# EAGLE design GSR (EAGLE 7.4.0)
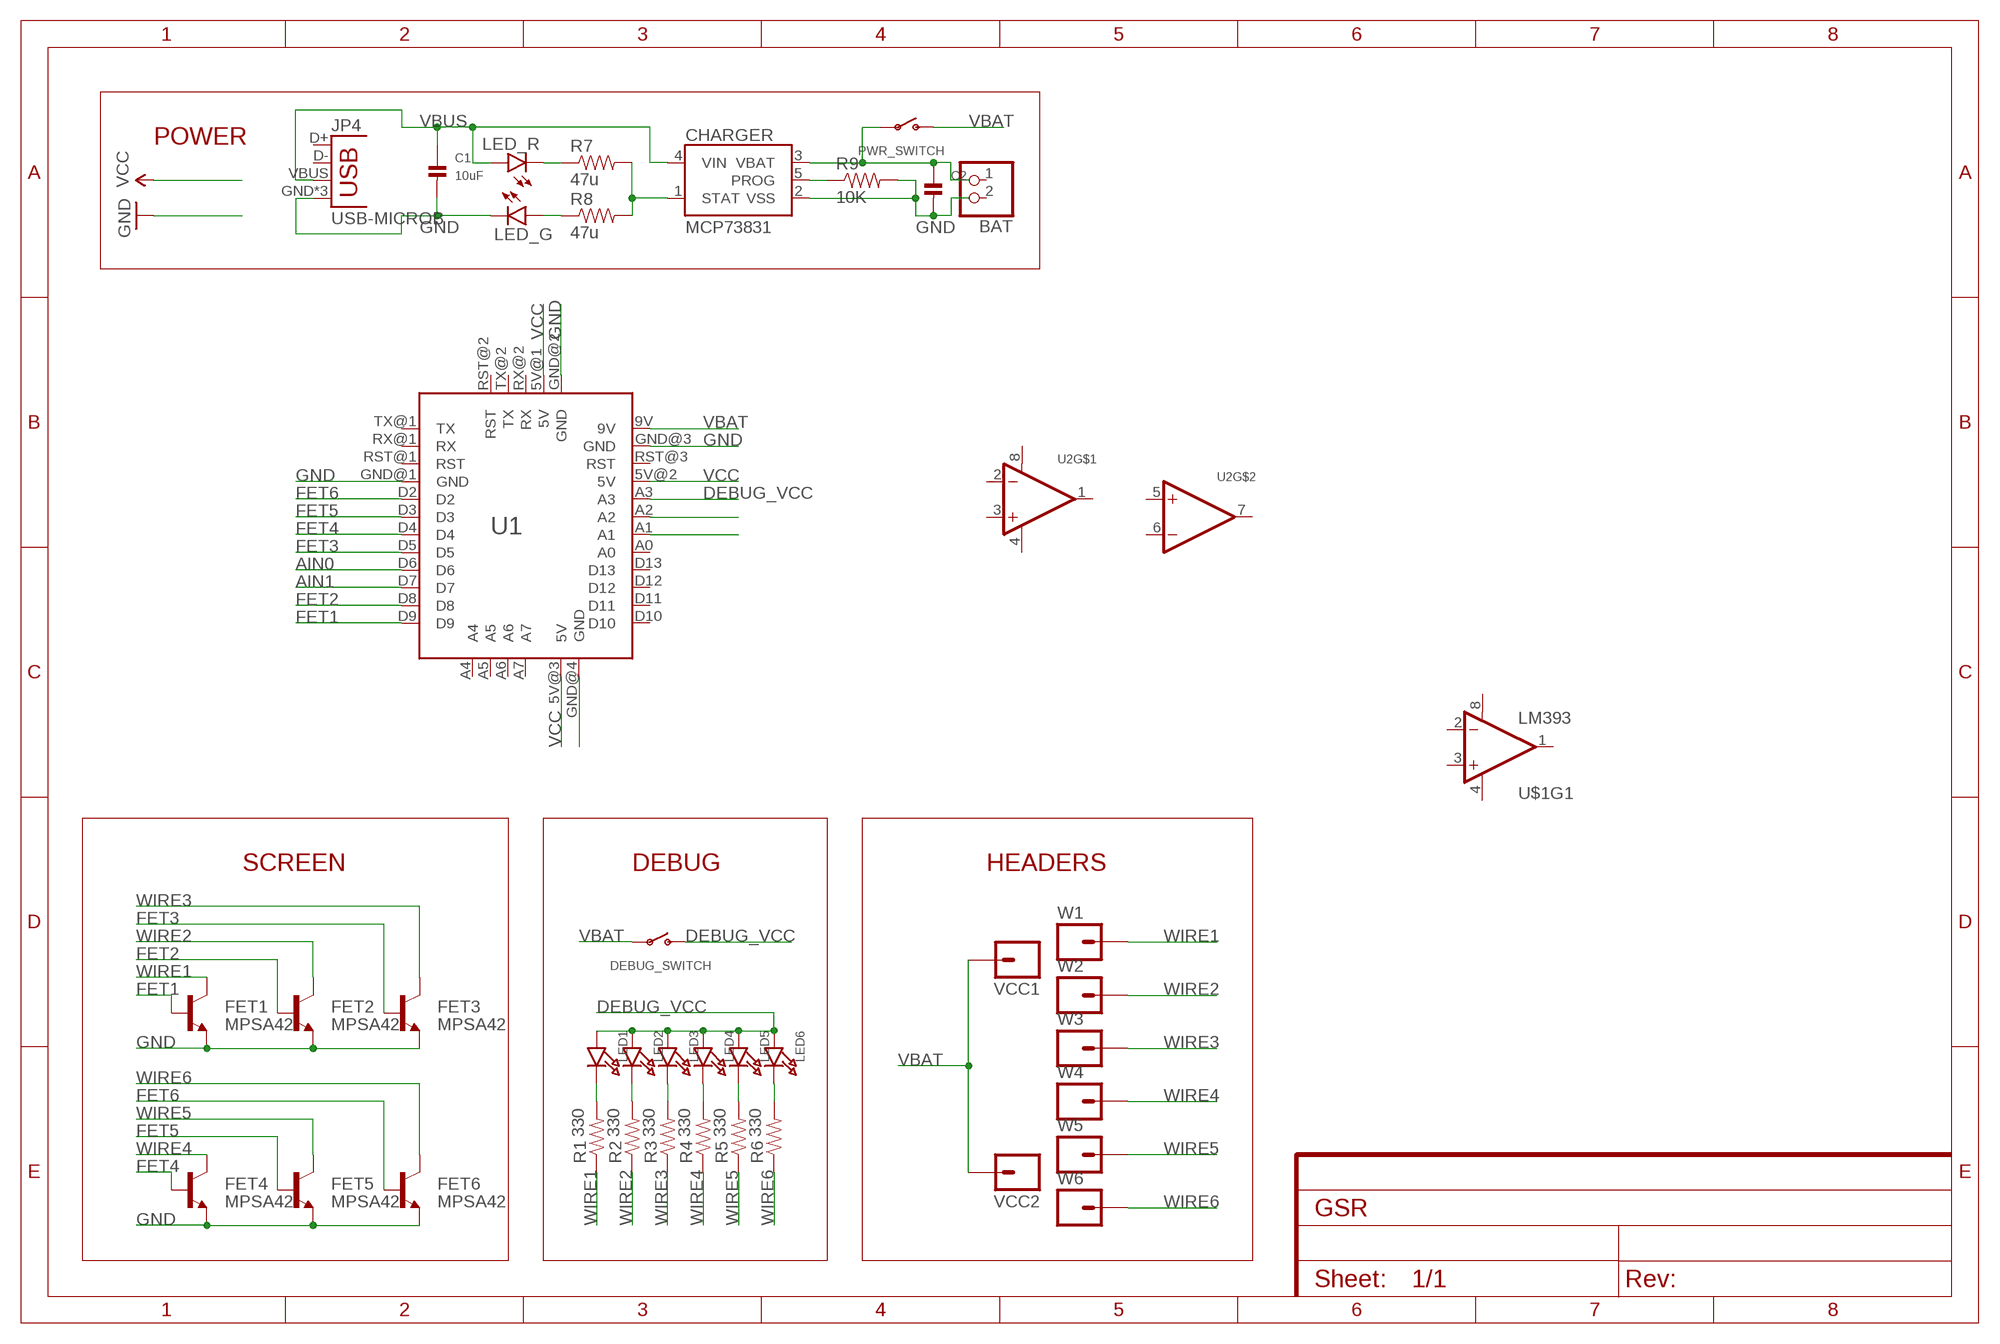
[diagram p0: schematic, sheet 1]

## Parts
BAT  JST_2PIN-SMT  [JST-PH-2-SMT]
C1  10uF  CAP_CERAMIC0603  [0603]
C2  CAP_CERAMIC0603  [0603]
CHARGER  MCP73831  [SOT23-5]
DEBUG_SWITCH  SWITCH_SPST  [SPST_SMT_19192]
FET1  MPSA42  TRANSISTOR_NPNMPSA42  [SOT23-3]
FET2  MPSA42  TRANSISTOR_NPNMPSA42  [SOT23-3]
FET3  MPSA42  TRANSISTOR_NPNMPSA42  [SOT23-3]
FET4  MPSA42  TRANSISTOR_NPNMPSA42  [SOT23-3]
FET5  MPSA42  TRANSISTOR_NPNMPSA42  [SOT23-3]
FET6  MPSA42  TRANSISTOR_NPNMPSA42  [SOT23-3]
JP4  USB-MICROB  [USB-MICROB]
LED1  LED0603_NOOUTLINE  [CHIPLED_0603_NOOUTLINE]
LED2  LED0603_NOOUTLINE  [CHIPLED_0603_NOOUTLINE]
LED3  LED0603_NOOUTLINE  [CHIPLED_0603_NOOUTLINE]
LED4  LED0603_NOOUTLINE  [CHIPLED_0603_NOOUTLINE]
LED5  LED0603_NOOUTLINE  [CHIPLED_0603_NOOUTLINE]
LED6  LED0603_NOOUTLINE  [CHIPLED_0603_NOOUTLINE]
LED_G  LED0603  [LED-0603]
LED_R  LED0603  [LED-0603]
PWR_SWITCH  SWITCH_SPST  [SPST_SMT_19192]
R1  330  RESISTOR0603-RES  [0603-RES]
R2  330  RESISTOR0603-RES  [0603-RES]
R3  330  RESISTOR0603-RES  [0603-RES]
R4  330  RESISTOR0603-RES  [0603-RES]
R5  330  RESISTOR0603-RES  [0603-RES]
R6  330  RESISTOR0603-RES  [0603-RES]
R7  47u  RESISTOR0603  [0603-RES]
R8  47u  RESISTOR0603  [0603-RES]
R9  10K  RESISTOR0603  [0603-RES]
U1  ARDUINO_MINI  [ARDUINO_MINI]
U2  OPAMP_DUALMSOP8_65  [MSOP8_0.65MM]
U$1  LM393  [SO08]
VCC1  M01NOSILK-KIT  [1X01NS-KIT]
VCC2  M01NOSILK-KIT  [1X01NS-KIT]
W1  M01NOSILK-KIT  [1X01NS-KIT]
W2  M01NOSILK-KIT  [1X01NS-KIT]
W3  M01NOSILK-KIT  [1X01NS-KIT]
W4  M01NOSILK-KIT  [1X01NS-KIT]
W5  M01NOSILK-KIT  [1X01NS-KIT]
W6  M01NOSILK-KIT  [1X01NS-KIT]

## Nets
AIN0: U1.D6
AIN1: U1.D7
DEBUG_VCC: DEBUG_SWITCH.C(S) LED1.A LED2.A LED3.A LED4.A LED5.A LED6.A U1.A3
FET1: FET1.1(B) U1.D9
FET2: FET2.1(B) U1.D8
FET3: FET3.1(B) U1.D5
FET4: FET4.1(B) U1.D4
FET5: FET5.1(B) U1.D3
FET6: FET6.1(B) U1.D2
GND: C1.2 C2.2 CHARGER.2(VSS) FET1.2(E) FET2.2(E) FET3.2(E) FET4.2(E) FET5.2(E) FET6.2(E) JP4.GND JP4.MT1(GND) JP4.MT2(GND) LED_G.C R9.2 U1.GND@1(GND) U1.GND@2(GND) U1.GND@3(GND) U1.GND@4(GND)
N$1: LED1.C R1.2
N$2: LED2.C R2.2
N$3: LED3.C R3.2
N$4: LED4.C R4.2
N$5: LED5.C R5.2
N$6: LED6.C R6.2
N$7: CHARGER.1(STAT) R7.2 R8.2
N$10: LED_G.A R8.1
N$11: LED_R.C R7.1
N$14: CHARGER.5(PROG) R9.1
N$36: U1.A2
N$37: U1.A1
VBAT: DEBUG_SWITCH.B(P) PWR_SWITCH.C(S) U1.9V VCC1.1 VCC2.1
VBAT_IN: C2.1 CHARGER.3(VBAT) PWR_SWITCH.B(P)
VBUS: C1.1 CHARGER.4(VIN) JP4.VBUS LED_R.A
VCC: U1.5V@1(5V) U1.5V@2(5V) U1.5V@3(5V)
WIRE1: FET1.3(C) R1.1 W1.1
WIRE2: FET2.3(C) R2.1 W2.1
WIRE3: FET3.3(C) R3.1 W3.1
WIRE4: FET4.3(C) R4.1 W4.1
WIRE5: FET5.3(C) R5.1 W5.1
WIRE6: FET6.3(C) R6.1 W6.1
Unconnected: BAT.1 BAT.2 JP4.D+ JP4.D- U1.A0 U1.A4 U1.A5 U1.A6 U1.A7 U1.D10 U1.D11 U1.D12 U1.D13 U1.RST@1(RST) U1.RST@2(RST) U1.RST@3(RST) U1.RX@1(RX) U1.RX@2(RX) U1.TX@1(TX) U1.TX@2(TX) U2.1(OUT) U2.2(-IN) U2.3(+IN) U2.5(+IN) U2.6(-IN) U2.7(OUT) U$1.1(OUT) U$1.2(-IN) U$1.3(+IN) U$1.5(+IN) U$1.6(-IN) U$1.7(OUT)

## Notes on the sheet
- POWER
- SCREEN | DEBUG | HEADERS

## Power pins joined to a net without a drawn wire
V+: U2.8(V+) U$1.8(V+)
V-: U2.4(V-) U$1.4(V-)

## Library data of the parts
BAT = adafruit:JST_2PIN: JST 2-Pin Connectors of various flavors
C1 C2 = microbuilder:CAP_CERAMIC: Ceramic Capacitors
CHARGER = SparkFun-PowerIC:MCP73831: Miniature single cell, fully integrated Li-Ion, Li-polymer charge management controller http://ww1.microchip.com/downloads/en/DeviceDoc/20001984g.pdf IC-09995; PROD_ID: IC-09995
DEBUG_SWITCH PWR_SWITCH = microbuilder:SWITCH_SPST: Switch - SPST
FET1-FET6 = SparkFun-DiscreteSemi:TRANSISTOR_NPN: Generic NPN BJT MMBT2222A - TRANS-08049 (SOT-23, 1A 40V) MPSA42 - TRANS-09116 (SOT-23, 500mA 300V) MMBT5088LT1G - TRANS-11160 (SOT-23, 50 mA 30V) BC547 - COM-08928 (TO-92 45V 100mA) (1.Collector 2.Base 3.Emitter) 2N3904 - COM-00521 (TO-92 40V 200mA) (1.Emitter 2.Base 3.Collector) P2N2222A -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; PROD_ID: TRANS-09116
JP4 = SparkFun-Connectors:USB: USB Connectors USB-B-PTH is fully proven SKU : PRT-00139/CONN-08278 USB-miniB is fully proven SKU : PRT-00587 USB-A-PCB is untested. USB-A-H is throughly reviewed, but untested. Spark Fun Electronics SKU : PRT-00437 USB-B-SMT is throughly reviewed, but untested. Needs silkscreen touching up.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; PROD_ID: CONN-09505
LED1-LED6 = microbuilder:LED: LED
LED_G LED_R = SparkFun-LED:LED: LEDs
R1-R6 = SparkFun-Passives:RESISTOR: Resistor
R7-R9 = SparkFun-Resistors:RESISTOR: Resistor
U1 = myParts:ARDUINO_MINI: Arduino Mini V5 Footprint
U2 = microbuilder:OPAMP_DUAL: Dual Op-Amp MSOP8 - 0.65mm Pitch Manuf. ID Slew Rate Gain Bandwidth Prod. -3dB Bandwidth Current Input Bias Voltage Input Offset Supply - Single Supply - Dual Digikey Mouser EL5236IYZ-T7 128V/µs 300MHz 250MHz 6.5µA 100µV 5-12V +/-2.5-6V EL5236IYZ-T7TR-ND --
U$1 = SparkFun-AnalogIC:LM393: Low-voltage comparator
VCC1 VCC2 W1-W6 = SparkFun-Connectors:M01: Header 1

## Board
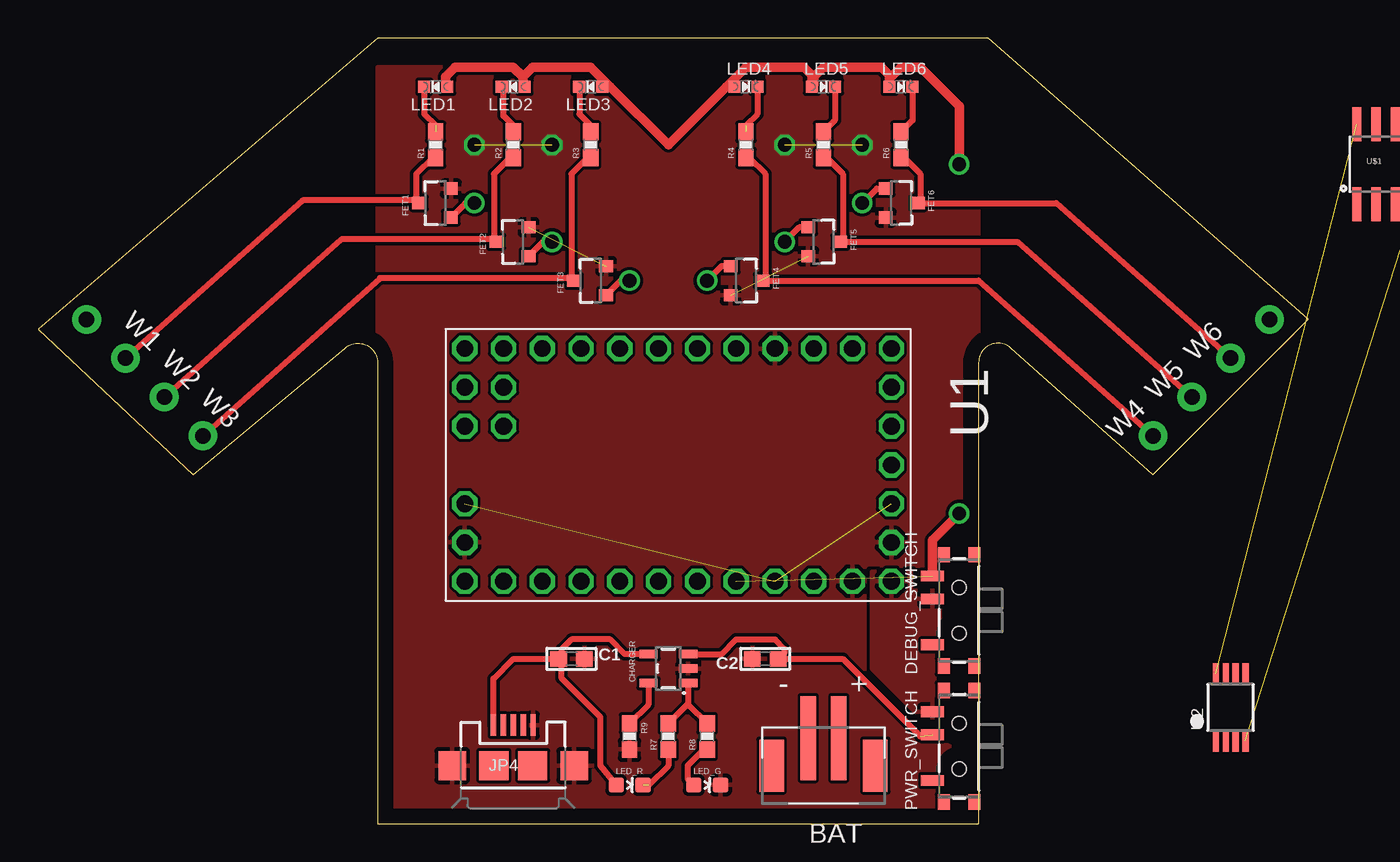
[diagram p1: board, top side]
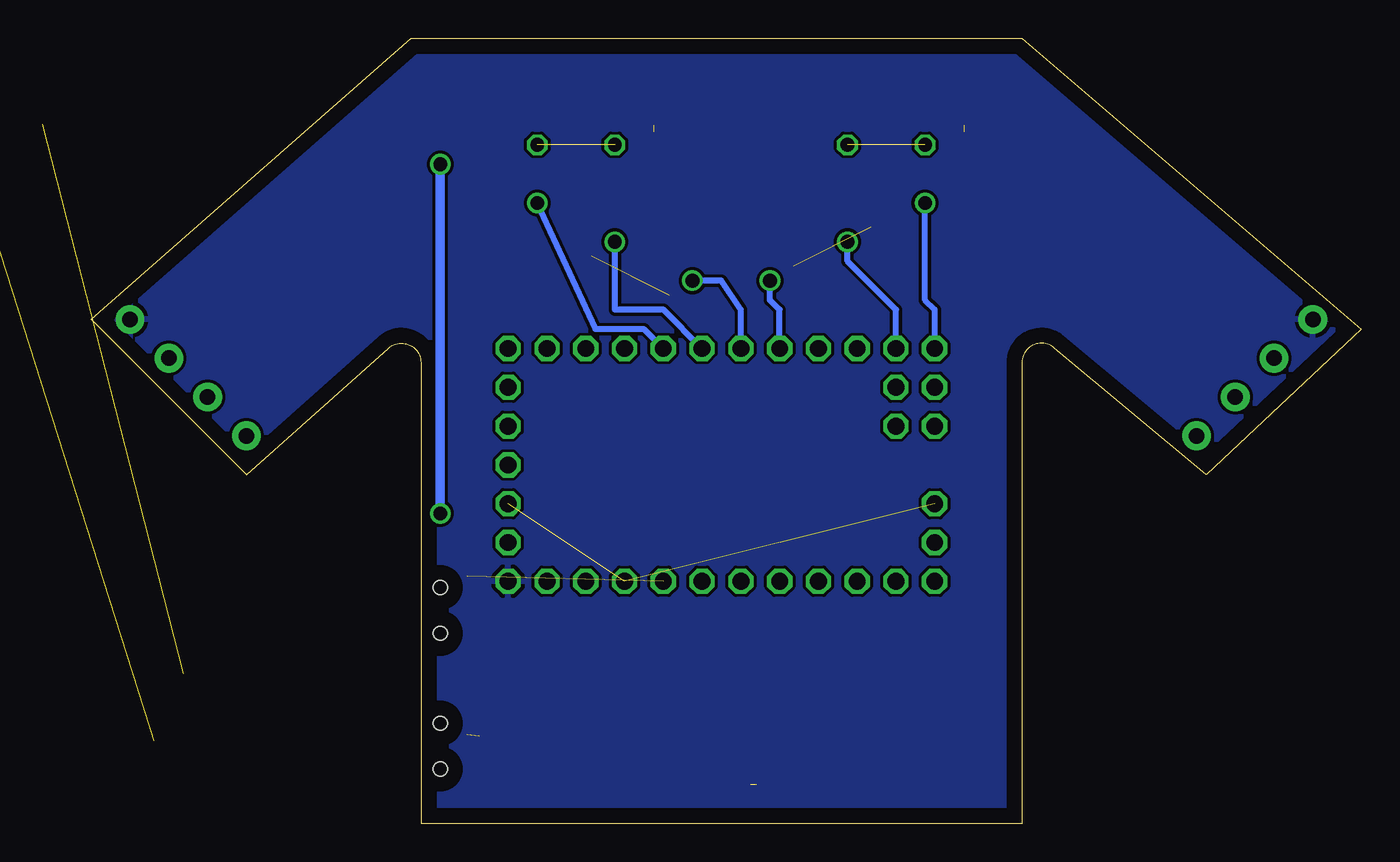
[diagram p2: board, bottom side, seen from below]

Size 83.19 x 51.44 mm. Coordinates in mm from the lower left corner, seen from the top.
Outline: 10.16,22.86 20.11,31.14 arc-132 22.22,30.19 22.22,0 61.59,0 61.59,30.19 arc-132 63.71,31.14 73.03,22.86 83.19,33.02 62.23,51.44 22.22,51.44 0,32.38 10.16,22.86
Copper layers (1*16): Top 0.035mm / dielectric 1.5mm / Bottom 0.035mm
Design rules "default": minimum track width 10mil, minimum drill 24mil, track to track 8mil, track to pad 8mil, pad to pad 8mil, via to via 8mil, smd to smd 8mil, copper to edge 40mil, drill to drill 8mil, minimum pad ring 10mil, minimum via ring 8mil, stop-mask expansion 4mil, vias tented up to drill 0mil, thermal gap 10mil

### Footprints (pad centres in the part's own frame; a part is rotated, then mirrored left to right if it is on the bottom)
JST-PH-2-SMT = smd 1 x 5.5: 1 -1,-1.8; 2 1,-1.8 | smd 1.6 x 3.4: NC1 -3.4,0; NC2 3.4,0
0603 = smd 1.1 x 1: 1 -0.85,0; 2 0.85,0
SOT23-5 = smd 0.55 x 1.2: 1 -0.95,-1.3; 2 0,-1.3; 3 0.95,-1.3; 4 0.95,1.3; 5 -0.95,1.3
SPST_SMT_19192 = smd 0.7 x 1.5: A -2.25,1.75; B 0.75,1.75; C 2.25,1.75 | smd 1 x 0.8: GND1 -3.65,1; GND2 -3.65,-1; GND3 3.65,1; GND4 3.65,-1 | hole 0.9: -1.5,0; 1.5,0
SOT23-3 = smd 0.8 x 0.9: 1 -0.95,-1; 2 0.95,-1; 3 0,1.1
USB-MICROB = smd 0.35 x 1.4: D+ 0,2.65; D- -0.65,2.65; GND 1.3,2.65; ID 0.65,2.65; VBUS -1.3,2.65 | smd 1.8 x 1.9: MT1 -4,0; MT2 4,0 | smd 1.9 x 1.9: P$1 -1.27,0; P$2 1.27,0
CHIPLED_0603_NOOUTLINE = smd 0.8 x 0.8: A 0,-0.75; C 0,0.75
LED-0603 = smd 1 x 1: A 0,-0.877; C 0,0.877
0603-RES = smd 1.1 x 1: 1 -0.85,0; 2 0.85,0
ARDUINO_MINI = drill 1.1 octagon: 5V@1 2.54,15.24; 5V@2 7.62,7.62; 5V@3 2.54,-12.7; 9V 7.62,15.24; A0 7.62,-2.54; A1 7.62,0; A2 7.62,2.54; A3 7.62,5.08; A4 -5.08,-12.7; A5 -2.54,-12.7; A6 -5.08,-10.16; A7 -2.54,-10.16; D2 -7.62,5.08; D3 -7.62,2.54; D4 -7.62,0; D5 -7.62,-2.54; D6 -7.62,-5.08; D7 -7.62,-7.62; D8 -7.62,-10.16; D9 -7.62,-12.7; D10 7.62,-12.7; D11 7.62,-10.16; D12 7.62,-7.62; D13 7.62,-5.08; GND@1 -7.62,7.62; GND@2 5.08,15.24; GND@3 7.62,12.7; GND@4 5.08,-12.7; RST@1 -7.62,10.16; RST@2 -5.08,15.24; RST@3 7.62,10.16; RX@1 -7.62,12.7; RX@2 0,15.24; TX@1 -7.62,15.24; TX@2 -2.54,15.24
MSOP8_0.65MM = smd 0.4 x 1.4: 1 -0.975,-2.2; 2 -0.325,-2.2; 3 0.325,-2.2; 4 0.975,-2.2; 5 0.975,2.2; 6 0.325,2.2; 7 -0.325,2.2; 8 -0.975,2.2
SO08 = smd 0.61 x 2.21: 1 -1.905,-2.616; 2 -0.635,-2.616; 3 0.635,-2.616; 4 1.905,-2.616; 5 1.905,2.616; 6 0.635,2.616; 7 -0.635,2.616; 8 -1.905,2.616
1X01NS-KIT = drill 1.016 pad 1.88: 1 0,0

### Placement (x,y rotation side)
BAT  51.44,3.81 180 top
C1  34.93,10.79 0 top
C2  47.62,10.79 180 top
CHARGER  41.28,10.16 90 top
DEBUG_SWITCH  60.33,13.97 90 top
FET1  26.04,40.64 90 top
FET2  31.11,38.1 90 top
FET3  36.2,35.56 90 top
FET4  46.36,35.56 270 top
FET5  51.44,38.1 270 top
FET6  56.52,40.64 270 top
JP4  31.11,3.81 0 top
LED1  26.04,48.26 90 top
LED2  31.11,48.26 90 top
LED3  36.2,48.26 90 top
LED4  46.36,48.26 270 top
LED5  51.44,48.26 270 top
LED6  56.52,48.26 270 top
LED_G  43.82,2.54 270 top
LED_R  38.73,2.54 270 top
PWR_SWITCH  60.33,5.08 90 top
R1  26.04,44.45 90 top
R2  31.11,44.45 90 top
R3  36.2,44.45 90 top
R4  46.36,44.45 90 top
R5  51.44,44.45 90 top
R6  56.52,44.45 90 top
R7  41.28,5.71 90 top
R8  43.82,5.71 90 top
R9  38.73,5.71 270 top
U1  40.64,23.5 270 top
U2  78.11,7.62 0 top
U$1  not placed on the board
VCC1  3.17,33.02 0 top
VCC2  80.64,33.02 0 top
W1  5.72,30.48 0 top
W2  8.25,27.94 0 top
W3  10.8,25.4 0 top
W4  73.03,25.4 0 top
W5  75.56,27.94 0 top
W6  78.11,30.48 0 top

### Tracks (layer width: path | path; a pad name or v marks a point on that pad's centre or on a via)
DEBUG_VCC  (via drill 0.9)  (1 unrouted)
  Top 0.406: LED6.A 55.77,48.78
  Top 0.61: DEBUG_SWITCH.C 58.58,18.57 v60.33,20.32 | v60.33,43.18 60.33,46.99 57.79,49.53 56.52,49.53 55.77,48.78 | LED6.A 55.77,49.01 55.25,49.53 51.44,49.53 50.8,48.9 50.8,48.38 LED5.A 50.69,49.01 50.17,49.53 46.36,49.53 45.09,48.26 | 45.09,48.26 41.28,44.45 37.47,48.26 | 31.75,48.9 32.39,49.53 36.2,49.53 37.47,48.26 | 31.75,48.9 31.11,49.53 27.3,49.53 26.67,48.9 26.67,48.38 LED1.A | 31.75,48.9 31.75,48.38 LED2.A | 37.47,48.26 LED3.A | LED4.A 45.09,48.26
  Bottom 0.61: v60.33,20.32 v60.33,43.18
FET1  (via drill 0.9)
  Top 0.406: v28.57,40.64 27.98,40.64 FET1.1
  Bottom 0.406: U1.D9 27.94,33.66 28.57,34.29 v28.57,40.64
FET2  (via drill 0.9)
  Top 0.406: v33.66,38.1 33.07,38.1 FET2.1
  Bottom 0.406: U1.D8 30.48,33.66 33.66,36.83 v33.66,38.1
FET3  (via drill 0.9)
  Top 0.406: v38.73,35.56 38.15,35.56 FET3.1
  Bottom 0.406: U1.D5 38.1,33.66 38.73,34.29 v38.73,35.56
FET4  (via drill 0.9)
  Top 0.406: FET4.1 44.77,36.51 v43.82,35.56
  Bottom 0.406: U1.D4 40.64,33.66 41.91,35.56 v43.82,35.56
FET5  (via drill 0.9)
  Top 0.406: FET5.1 49.85,39.05 v48.9,38.1
  Bottom 0.406: U1.D3 45.72,33.66 48.9,33.66 v48.9,38.1
FET6  (via drill 0.9)
  Top 0.406: v53.98,40.64 54.93,41.59 FET6.1
  Bottom 0.406: U1.D2 46.99,32.38 50.17,32.38 v53.98,40.64
GND  (via drill 0.9)  (4 unrouted)
  other vias: 28.57,44.45 33.66,44.45 48.9,44.45 53.98,44.45
  pour Top (rank 2): 22.22,0 61.59,0 61.59,49.53 22.22,49.53
N$1  (1 unrouted)
  Top 0.406: LED1.C 25.29,46.47 26.04,45.72
N$2
  Top 0.406: R2.2 31.11,45.72 30.48,46.36 30.48,48.15 LED2.C
N$3
  Top 0.406: LED3.C 35.45,46.47 36.2,45.72 R3.2
N$4  (1 unrouted)
  Top 0.406: LED4.C 47.11,46.47 46.36,45.72
N$5
  Top 0.406: LED5.C 52.19,46.05 R5.2
N$6
  Top 0.406: LED6.C 57.27,46.05 R6.2
N$7
  Top 0.406: R7.2 42.58,7.87 CHARGER.1 42.58,7.8 R8.2
N$8
  Top 0: 83.19,33.02 81.28,31.12
N$10
  Top 0.406: R8.1 43.82,5.08 42.55,3.81 42.55,2.93 LED_G.A
N$11  (1 unrouted)
  Top 0.406: R7.1 41.28,3.81 40.01,2.54
N$14
  Top 0.406: CHARGER.5 39.98,7.8 R9.1
V+  (1 unrouted)
V-  (1 unrouted)
VBAT
  pour Bottom: -3.17,52.07 90.81,52.07 92.08,-20.32 -3.17,-20.32
  pour Top: 54.61,16.51 57.15,16.51 57.15,15.24 59.05,15.24 59.05,6.98 57.79,6.98 54.61,10.16
VBAT_IN  (1 unrouted)
  Top 0.406: 57.79,5.71 52.71,10.79 C2.1 48.9,11.21 48.9,11.43 48.26,12.06 45.72,12.06 44.77,11.11 CHARGER.3
VBUS
  Top 0.406: JP4.VBUS 29.82,9.49 31.11,10.79 C1.1 | LED_R.A 36.83,3.81 36.83,6.98 34.29,9.53 34.29,11.21 C1.1 | CHARGER.4 38.42,11.11 37.47,12.06 34.93,12.06 34.29,11.43 34.29,11.01 C1.1
VCC  (2 unrouted)
WIRE1
  Top 0.406: R1.1 25.82,43.6 24.77,42.55 24.77,40.81 | 24.77,40.81 FET1.3 | 24.77,40.81 17.31,40.81 W1.1
WIRE2
  Top 0.406: R2.1 30.9,43.6 29.85,42.55 29.85,38.27 | 29.85,38.27 FET2.3 | 29.85,38.27 19.86,38.27 W2.1
WIRE3
  Top 0.406: R3.1 35.98,43.6 34.93,42.55 34.93,35.73 | 34.93,35.73 FET3.3 | 34.93,35.73 22.39,35.73 W3.1
WIRE4
  Top 0.406: W4.1 61.59,35.56 FET4.3 47.62,35.73 47.62,42.55 46.57,43.6 R4.1
WIRE5
  Top 0.406: W5.1 64.14,38.1 FET5.3 52.71,38.27 52.71,42.55 51.65,43.6 R5.1
WIRE6
  Top 0.406: W6.1 66.67,40.64 FET6.3 57.79,40.81 57.79,42.55 56.73,43.6 R6.1

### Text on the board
tSilk: W6 | W1 | W5 | W2 | W4 | W3

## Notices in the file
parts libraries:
SparkFun-Aesthetics: Licensing: Creative Commons ShareAlike 4.0 International - https://creativecommons.org/licenses/by-sa/4.0
microbuilder: This work is placed in the public domain, and may be freely used for commercial and non-commercial work with the following conditions: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
